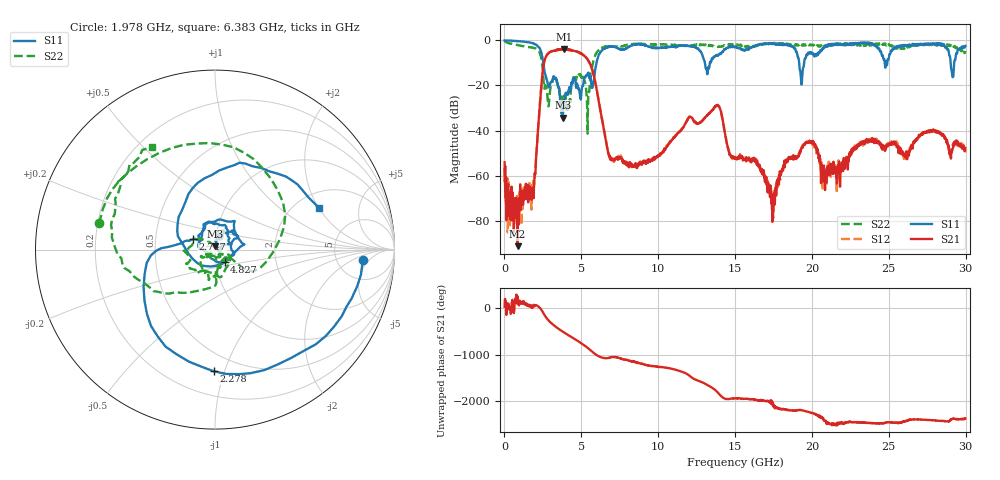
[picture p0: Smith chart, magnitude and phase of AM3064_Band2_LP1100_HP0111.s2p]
# Hz S DB R 50.0
!freq dBS11 angS11 dBS21 angS21 dBS12 angS12 dBS22 angS22
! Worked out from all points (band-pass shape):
!   1600 points, 10 MHz to 29.98 GHz, reference 50 ohm
!   highest |S21| = -3.96 dB at 3.89 GHz (marker M1); lowest = -91.3 dB at 853.5 MHz (marker M2)
!   |S21| within 3 dB of the highest: 2.72 GHz to 5.214 GHz (2.494 GHz wide, 62.9 % of centre)
!   lowest |S11| = -34.2 dB at 3.796 GHz (marker M3), VSWR 1.04, Z = 50.2 + j1.94 ohm
!   |S11| at or under -10 dB: 2.529 GHz to 5.99 GHz (3.461 GHz wide, 81.2 % of centre); 13.04 GHz to 13.36 GHz (315.9 MHz wide, 2.39 % of centre); 19.17 GHz to 19.49 GHz (324.9 MHz wide, 1.68 % of centre)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
!   |S22| runs from -41.4 to -0.3 dB; largest |S21 - S12| = 0.021
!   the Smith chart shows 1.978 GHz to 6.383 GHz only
!   S11 on the Smith chart (normalised r, x): 1.978 GHz: 9.16, -3.42; 2.278 GHz: 0.37, -0.92; 2.747 GHz: 0.78, +0.09; 4.827 GHz: 1.10, -0.16; 6.383 GHz: 2.67, +2.00
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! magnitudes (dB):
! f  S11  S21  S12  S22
! 10 MHz  0.0  -54.0  -56.4  -0.3
! 853.5 MHz  -0.3  -91.3  -71.7  -2.0
! 1.978 GHz  -1.7  -59.0  -58.7  -3.6
! 2.278 GHz  -3.4  -30.9  -30.8  -5.2
! 2.747 GHz  -17.3  -6.7  -6.6  -21.8
! 3.796 GHz  -34.2  -4.0  -3.9  -27.3
! 3.89 GHz  -26.6  -4.0  -4.0  -25.7
! 4.827 GHz  -21.1  -5.3  -5.2  -15.2
! 5.015 GHz  -22.0  -6.0  -6.0  -16.6
! 5.408 GHz  -14.8  -8.5  -8.4  -41.4
! 6.383 GHz  -4.1  -36.7  -36.6  -3.5
! 7.001 GHz  -2.9  -53.0  -52.6  -2.6
! 10 GHz  -3.4  -51.3  -51.1  -1.8
! 13.82 GHz  -6.5  -28.7  -28.8  -2.6
! 15 GHz  -2.8  -52.0  -52.2  -1.9
! 17.52 GHz  -1.5  -68.0  -71.9  -1.2
! 19.33 GHz  -19.6  -47.3  -48.1  -2.2
! 19.99 GHz  -5.4  -45.0  -45.2  -1.9
! 20.83 GHz  -3.1  -58.0  -57.9  -2.3
! 25 GHz  -8.0  -46.2  -46.6  -1.7
! 29.18 GHz  -16.2  -47.7  -46.5  -2.3
! 29.98 GHz  -2.4  -47.8  -49.7  -4.8
